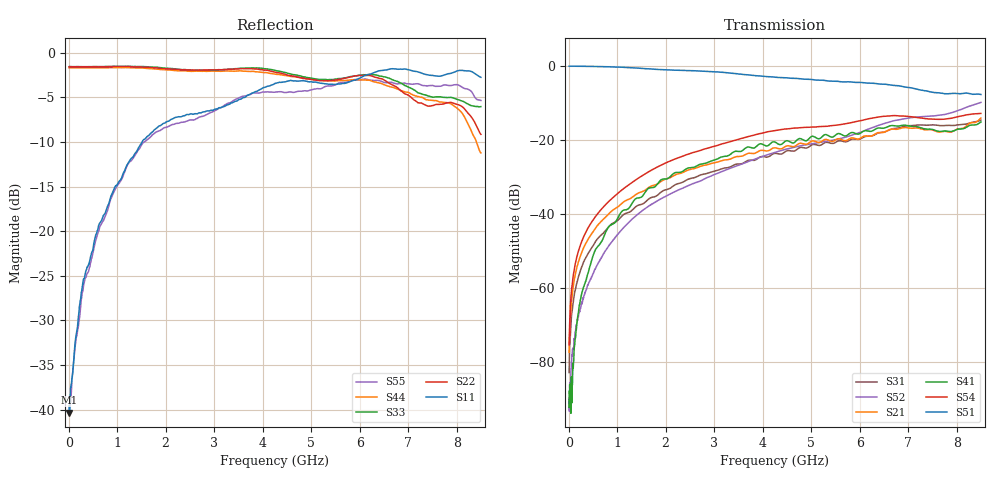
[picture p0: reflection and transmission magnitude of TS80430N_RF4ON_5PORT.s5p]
!Created with skrf (http://scikit-rf.org).
# GHz S RI R 50.0
!freq ReS11 ImS11 ReS12 ImS12 ReS13 ImS13
! ReS14 ImS14 ReS15 ImS15
! ReS21 ImS21 ReS22 ImS22 ReS23 ImS23
! ReS24 ImS24 ReS25 ImS25
! ReS31 ImS31 ReS32 ImS32 ReS33 ImS33
! ReS34 ImS34 ReS35 ImS35
! ReS41 ImS41 ReS42 ImS42 ReS43 ImS43
! ReS44 ImS44 ReS45 ImS45
! ReS51 ImS51 ReS52 ImS52 ReS53 ImS53
! ReS54 ImS54 ReS55 ImS55
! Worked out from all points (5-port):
!   1601 points, 10 MHz to 8.5 GHz, reference 50 ohm
!   strongest paths, dB at 10 MHz, 2.132 GHz, 4.255 GHz, 6.378 GHz, 8.5 GHz:
!     S51: -0.1, -1.2, -3.1, -4.9, -7.8
!     S54: -75.2, -25.5, -17.5, -13.9, -12.9
!     S41: -87.8, -29.4, -20.6, -16.8, -15.2
!     S21: -77.2, -29.9, -22.1, -18.0, -14.1
!     S52: -89.6, -34.3, -23.4, -16.1, -9.9
!     S31: -82.7, -32.7, -23.6, -18.2, -14.7
!   lowest |S11| = -40.3 dB at 15.31 MHz (marker M1), VSWR 1.02, Z = 50.9 - j0.317 ohm
!   |S11| at or under -10 dB: start of sweep to 1.512 GHz
